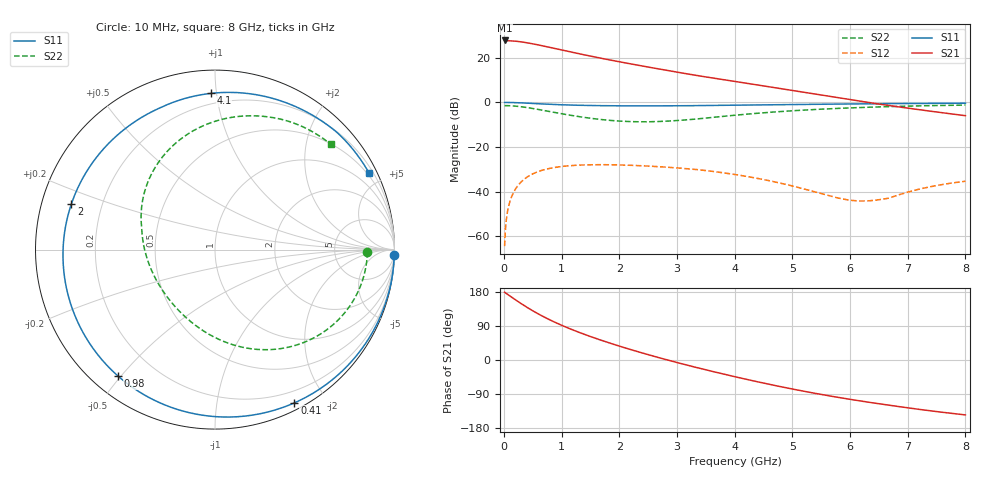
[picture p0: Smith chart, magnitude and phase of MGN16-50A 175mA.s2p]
! Port[1] = GATE
! Port[2] = DRAIN
! [Type]  S-parameter s2p file touchstone ver. 1.0
! [Object]  MGN16-50A
! [Bias]  175 mA
! [Version]  1.0
! [Date]  Thu May 28 11:04:00 2026
! [Source]  This file was created in JSC "ICC Milandr".
! [Disclaimer] Property of JSC "ICC Milandr". Unauthorized reproduction and/or distribution is strictly prohibited.
!  The file and the data are provided "AS IS" and with all faults and disclaim all warranties, express and implied, including
!  without limitation any implied warranties of merchantability, fitness for a particular purpose.
!  JSC "ICC Milandr" assumes no liability for:
!  1) the accuracy of the data provided;
!  2) the proper functioning of this data;
!  3) infringement of patents, copyrights or intellectual property rights resulting from the use of this data.
!  JSC "ICC Milandr" reserves the right to make changes to the products and the data without prior notice.
!  Please, be aware that your receipt and use of the file provided shall serve as acceptance of these terms and conditions.
!  If you do not accept these terms, you should return or destroy this file and any other accompanying information immediately.
# hz S ma R 12.5
! 2 Port Network Data from SP1.SP block
! freq  magS11  angS11  magS21  angS21  magS12  angS12  magS22  angS22
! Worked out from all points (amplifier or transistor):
!   800 points, 10 MHz to 8 GHz, reference 12.5 ohm
!   highest |S21| = 27.8 dB at 10 MHz (marker M1)
!   |S21| within 3 dB of that: start of sweep to 775.7 MHz
!   unconditionally stable (mu >= 1): 4.186 GHz to end of sweep
!   at 1.34 GHz: K = 0.19, MSG = 24.8 dB, |S12| = -28.0 dB
!   at 4.01 GHz: K = 0.91, MSG = 20.8 dB, |S12| = -32.3 dB
!   at 8 GHz: K = 1.05, MAG = 13.3 dB, |S12| = -35.3 dB
!   S11 on the Smith chart (normalised r, x): 10 MHz: 2, -72; 410 MHz: 0.07, -1.64; 980 MHz: 0.07, -0.49; 2 GHz: 0.09, +0.15; 4.1 GHz: 0.13, +0.96; 8 GHz: 0.40, +4.24
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1e7  0.9992 -1.6  24.42 178.8  0.0006036 82.0  0.8488 -0.9
4e7  0.9988 -6.5  24.33 175.6  0.002387 84.0  0.8482 -3.7
9e7  0.997 -14.5  24.18 170.2  0.005335 79.9  0.8443 -8.4
1.8e8  0.9905 -28.7  23.69 160.7  0.01046 71.1  0.8302 -16.7
3e8  0.977 -46.9  22.69 148.5  0.01671 59.6  0.7997 -27.2
4.1e8  0.9617 -62.6  21.54 137.9  0.0217 49.5  0.7638 -36.2
5.3e8  0.944 -78.6  20.16 127.1  0.02625 39.3  0.7202 -45.4
6.6e8  0.9253 -94.4  18.62 116.3  0.03022 29.1  0.6719 -54.6
8.2e8  0.9047 -112.0  16.8 104.1  0.03389 17.6  0.6151 -65.0
9.8e8  0.8876 -127.6  15.13 92.9  0.03648 7.2  0.5637 -74.6
1.16e9  0.8724 -143.3  13.46 81.4  0.03843 -3.5  0.5138 -84.6
1.35e9  0.8603 -158.0  11.94 70.2  0.03964 -13.9  0.4702 -94.8
1.65e9  0.8475 -178.1  9.949 53.9  0.04032 -28.9  0.4186 -110.4
2e9  0.8396 162.3  8.131 36.6  0.0398 -44.9  0.3823 -128.6
2.33e9  0.8369 146.6  6.781 21.5  0.03846 -58.8  0.3687 -146.0
2.68e9  0.8379 132.3  5.631 6.4  0.03642 -72.8  0.3736 -164.4
3.27e9  0.8462 112.6  4.153 -17.3  0.03199 -95.0  0.4178 166.8
4.01e9  0.868 93.6  2.945 -44.3  0.02423 -113.0  0.5179 138.0
4.1e9  0.8707 91.5  2.825 -47.5  0.02322 -114.8  0.5306 134.8
5.34e9  0.9064 66.0  1.572 -86.5  0.01033 -124.7  0.6895 96.3
6.67e9  0.9418 44.3  0.8526 -119.1  0.007164 -69.3  0.806 65.5
8e9  0.9587 26.3  0.5049 -144.9  0.0172 -61.5  0.8718 42.4
